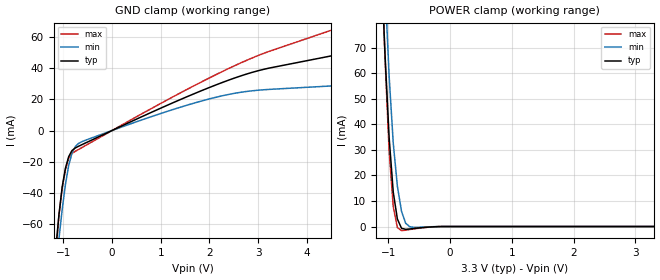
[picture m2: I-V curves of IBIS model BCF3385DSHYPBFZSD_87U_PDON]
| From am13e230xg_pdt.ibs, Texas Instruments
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|   Model BCF3385DSHYPBFZSD_87U_PDON
[Model] BCF3385DSHYPBFZSD_87U_PDON
Model_type Input
Polarity   Non-Inverting
Enable   Active-High
Vinl =  0.990V
Vinh =  2.310V
C_comp   0.593pF   0.545pF   0.644pF
[Model Spec]
Vinh   2.310V   2.079V   2.541V
Vinl   0.990V   0.891V   1.089V
[Temperature Range]   25.000   0.155k   -40.000
[Voltage Range]   3.300V   2.970V   3.630V
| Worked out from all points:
|   GND clamp passes 1 mA (typ) near -0.07 V on its own axis
|   POWER clamp passes 1 mA (typ) near -0.67 V on its own axis
[GND_clamp]
|Voltage   I(typ)   I(min)   I(max)
-3.3V     -1.011A    -884.9mA   -1.28A
-1.156V   -76.88mA   -90.37mA   -80.57mA
-1.089V   -54.34mA   -69.73mA   -54.73mA
-1.022V   -36.25mA   -50.83mA   -37.1mA
-955mV    -24.19mA   -34.63mA   -25.16mA
-888mV    -16.76mA   -22.37mA   -17.58mA
-821mV    -12.88mA   -14.56mA   -14.76mA
-754mV    -11.23mA   -10.35mA   -13.41mA
1.189V    17.02mA    12.89mA    20.64mA
2.328V    31.68mA    22.8mA     38.93mA
3.266V    40.44mA    26.55mA    51.4mA
6.6V      60.98mA    32.35mA    86.96mA
[POWER_clamp]
|Voltage   I(typ)   I(min)   I(max)
-3.3V     1.722A     1.973A     1.84A
-1.122V   107.2mA    137.2mA    110.5mA
-1.055V   67.72mA    94.79mA    66.44mA
-988mV    34.94mA    59.05mA    29.78mA
-921mV    13.45mA    32.66mA    7.761mA
-854mV    2.926mA    15.82mA    -428.8uA
-787mV    -691.9uA   5.965mA    -1.61mA
-720mV    -1.106mA   1.289mA    -1.422mA
-653mV    -960.7uA   -93.94uA   -1.168mA
-586mV    -772.5uA   -324.4uA   -929.9uA
-117mV    0A         0A         0A
3.3V      0A         0A         0A
